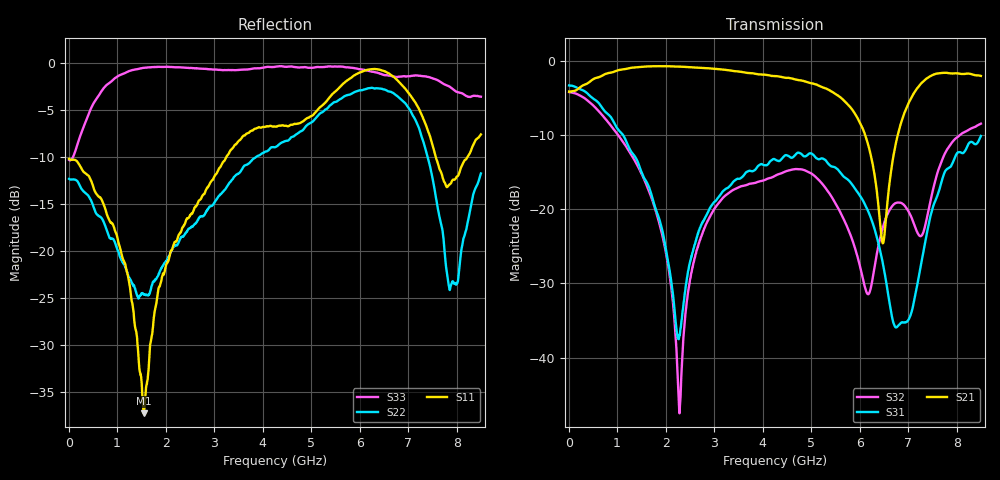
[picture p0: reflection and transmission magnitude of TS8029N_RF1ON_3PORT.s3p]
!Created with skrf (http://scikit-rf.org).
# GHz S RI R 50.0
!freq ReS11 ImS11 ReS12 ImS12 ReS13 ImS13
! ReS21 ImS21 ReS22 ImS22 ReS23 ImS23
! ReS31 ImS31 ReS32 ImS32 ReS33 ImS33
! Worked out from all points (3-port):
!   1601 points, 10 MHz to 8.5 GHz, reference 50 ohm
!   strongest paths, dB at 10 MHz, 2.132 GHz, 4.255 GHz, 6.378 GHz, 8.5 GHz:
!     S21: -4.1, -0.7, -2.0, -18.9, -2.0
!     S31: -3.3, -30.5, -13.3, -24.3, -10.1
!     S32: -4.2, -31.4, -15.5, -25.2, -8.4
!   lowest |S11| = -37.3 dB at 1.549 GHz (marker M1), VSWR 1.03, Z = 51.4 + j0.05 ohm
!   |S11| at or under -10 dB: start of sweep to 3.249 GHz; 7.571 GHz to 8.221 GHz (649.3 MHz wide, 8.22 % of centre)
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0.01  -0.3104 0.00654  0.6231 0.00265  0.6856 -0.012
      0.623 0.00261  -0.2427 0.00509  0.618 -0.012
      0.6854 -0.0121  0.6184 -0.012  -0.3053 0.0207
0.5671563  -0.1377 0.1489  0.7707 -0.00135  0.3529 -0.411
           0.7708 -0.00104  -0.0855 0.134  0.2862 -0.3852
           0.3528 -0.411  0.2861 -0.385  0.356 0.5366
1.548812  0.0137 0.000487  0.8271 -0.4002  -0.0421 -0.159
          0.8267 -0.3999  0.0554 -0.0195  -0.0785 -0.141
          -0.0422 -0.1588  -0.0787 -0.1412  0.8739 -0.3616
2.286381  -0.0436 -0.1157  0.6421 -0.6555  0.0115 -0.00847
          0.6425 -0.6549  -0.0644 -0.0944  -0.00188 0.00376
          0.0114 -0.00848  -0.00183 0.00379  0.4885 -0.8184
2.827619  -0.1354 -0.1616  0.4592 -0.7716  0.089 0.00877
          0.459 -0.7709  -0.1522 -0.0505  0.0771 0.0127
          0.089 0.0088  0.0773 0.0127  0.0598 -0.9335
4.255  -0.4361 -0.1499  -0.0951 -0.7876  0.1516 -0.1557
       -0.0952 -0.7865  -0.3341 0.1268  0.1044 -0.1316
       0.151 -0.1558  0.1047 -0.1317  -0.7968 -0.5333
6.467706  -0.3694 0.8385  -0.0256 -0.0544  -0.0426 -0.0143
          -0.0256 -0.0544  0.5311 0.5028  0.0648 -0.034
          -0.0427 -0.0143  0.0649 -0.034  -0.0872 0.8692
7.459975  0.2395 0.3222  -0.127 -0.7825  0.0181 0.0883
          -0.1257 -0.7819  0.1012 -0.2574  0.1107 -0.0266
          0.0182 0.0882  0.1107 -0.0271  0.8398 0.019
7.868556  0.0285 0.2264  -0.4614 -0.6859  0.1745 0.0832
          -0.4607 -0.6862  -0.0549 -0.0327  0.2171 -0.1655
          0.1742 0.0829  0.2169 -0.165  0.5581 -0.4982
8.5  -0.1187 0.4015  -0.6678 -0.4308  0.2964 -0.0992
     -0.6677 -0.4312  -0.1427 0.2166  0.115 -0.3602
     0.2965 -0.0995  0.1143 -0.3609  -0.3777 -0.5473
